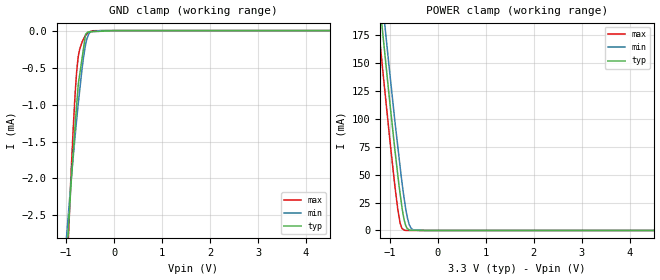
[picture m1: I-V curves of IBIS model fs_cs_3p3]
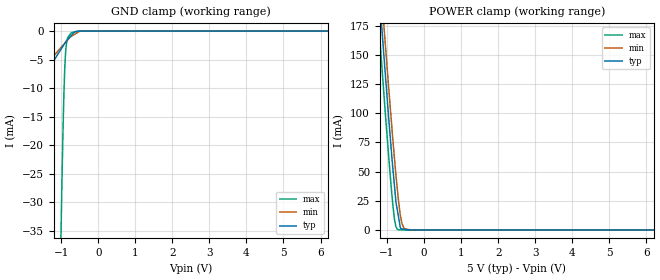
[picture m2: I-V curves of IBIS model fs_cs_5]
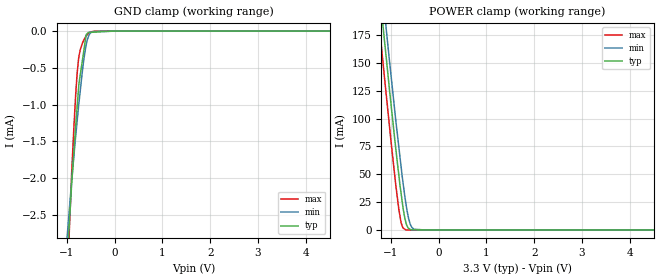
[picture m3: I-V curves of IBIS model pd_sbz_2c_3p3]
|Texas Instruments Incorporated
| 16-Bit 600KSPS Serial ADC with Ref and Pseudo Bipolar,
| Fully Differential Input
| Marketing part#   Digital Voltage Range   Package-type   #pins
| ADS8372IBRHPR   2.7V - 5.25V   VQFN   28
| ADS8372IBRHPRG4   2.7V - 5.25V   VQFN   28
| ADS8372IBRHPT   2.7V - 5.25V   VQFN   28
| ADS8372IBRHPTG4   2.7V - 5.25V   VQFN   28
| ADS8372IRHPR   2.7V - 5.25V   VQFN   28
| ADS8372IRHPRG4   2.7V - 5.25V   VQFN   28
| ADS8372IRHPT   2.7V - 5.25V   VQFN   28
| ADS8372IRHPTG4   2.7V - 5.25V   VQFN   28
[IBIS Ver]   3.2
[File name]   ads8372.ibs
|SIMDE Ver   V3.0 - 201101 - RHL4 - Build 457
[File Rev]   1.0
[Date]   6/17/2011
[Source]
| Texas Instruments Incorporated.
| Analog-eLab Design Center, HPA
| 12500 TI Blvd
| Dallas, TX -75243
| e-mail: elab_scm_ibis@list.ti.com
[Notes]   Revision History:
| Rev 1.0: 6/17/2011
| - Initial version of the model
| - Model generated from simulations in TISPICE
| - Model matched to SPICE simulation
| - C_comp although listed in numerical order of value are
|   obtained from varying PVT conditions. For PVT conditions for
|   each specific value refer the buffer description under
|   respective [Model]. IBIS model user is responsible for using
|   appropriate C_comp to simulate for Signal Integrity.
| - Model names with a trailing _3p3 contains the model for
|   3.3V [3.0V and 3.6V]. Model names with a trailing _5 contains
|   the model for 5.0V [4.75V and 5.25V].
| - SDO pin ibis is modeled in two modes of operation sdo_1drv_*
|   with single driver & sdo_2drv_* 2 driver blocks connected to SDO pad pin.
|   Inbuilt OR logic is used for mode selection.
| - Relative part of ADS8380.
[Disclaimer]
| This model is designed as an aid for customers of Texas Instruments.
| TI and its licensors and suppliers make no warranties, either expressed
| or implied, with respect to this  model, including the warranties of
| merchantability or fitness for a particular purpose. The model is
| provided solely on an "as is" basis. The entire risk as to its quality
| and performance is with the customer.
[Copyright]
 (C) Copyright 2011 Texas Instruments Incorporated.All rights reserved.
|   ADS8372
[Component]   ADS8372
[Manufacturer]   TI
[Package]   |28 VQFN   -  RHP package
|   typ   min   max
R_pkg   0.07673   0.07403   0.08176
L_pkg   1.23150nH   1.17718nH   1.32308nH
C_pkg   0.19965pF   0.19514pF   0.20511pF
[Pin]  signal_name   model_name   R_pin   L_pin   C_pin
1   AGND   GND   0.07820   1.25848nH  0.20073pF
2   AGND   GND   0.07674   1.23138nH  0.20002pF
3   +VA   POWER   0.07537   1.20618nH  0.19911pF
4   AGND   GND   0.07406   1.18248nH  0.19804pF
5   AGND   GND   0.07441   1.18988nH  0.19838pF
6   +VA   POWER   0.07613   1.22288nH  0.20045pF
7   REFM   GND   0.08029   1.30198nH  0.20374pF
8   REFIN   TERM   0.07725   1.24688nH  0.19750pF
9   REFOUT   TERM   0.07703   1.24278nH  0.19851pF
10   NC   NC   0.07445   1.19468nH  0.19621pF
11   +IN   TERM   0.07407   1.18748nH  0.19545pF
12   -IN   TERM   0.07475   1.20008nH  0.19514pF
13   NC   NC   0.00007   0.00128nH  0.12029pF
14   +VA   POWER   0.08623   1.41618nH  0.20518pF
15   AGND   GND   0.07587   1.21778nH  0.19615pF
16   +VA   POWER   0.07435   1.18858nH  0.19555pF
17   +VA   POWER   0.07401   1.18158nH  0.19546pF
18   AGND   GND   0.07505   1.20028nH  0.19719pF
19   AGND   GND   0.03811   0.83717nH  0.23761pF
20   +VBD   POWER   0.07794   1.25358nH  0.19975pF
21   BDGND   GND   0.07776   1.25028nH  0.19781pF
22   BUSY   BUSY   0.08176   1.32308nH  0.20511pF
23   SDO   SDO   0.07780   1.24828nH  0.20181pF
24   SCLK   SCLK_CONVEST   0.07628   1.21958nH  0.20091pF
25   _CONVST   SCLK_CONVEST   0.07403   1.17718nH  0.19891pF
26   _CS   FS_CS   0.07482   1.19198nH  0.19852pF
27   FS   FS_CS   0.07568   1.20828nH  0.20001pF
28   PD   PD_SBZ_2C   0.08058   1.30088nH  0.20427pF
29   THERMAL_PAD   NC   0.00007   0.00128nH  2.20537pF
|   Model Selectors
[Model Selector] FS_CS
fs_cs_3p3  3.3V digital input
fs_cs_5   5.0V digital input
[Model Selector] PD_SBZ_2C
pd_sbz_2c_3p3  3.3V digital input
pd_sbz_2c_5   5.0V digital input
[Model Selector] SCLK_CONVEST
sclk_convest_3p3  3.3V digital input
sclk_convest_5   5.0V digital input
[Model Selector] BUSY
busy_3p3  3.3V digital 3-state
busy_5   5.0V digital 3-state
[Model Selector] SDO
sdo_1drv_3p3  3.3V digital 3-state
sdo_1drv_5   5.0V digital 3-state
sdo_2drv_3p3  3.3V digital 3-state
sdo_2drv_5   5.0V digital 3-state
[Model Selector] TERM
term_3-3V  3.3V nominal termination
term_5-0V  5.0V nominal termination
[Model] term_3-3V
Model_type Terminator
C_comp   1.0e-20F  1.0e-20F  1.0e-20F
|   typ   min   max
[Voltage Range]   3.3V   3.0V   3.6V
[POWER Clamp Reference]   3.3V   3.0V   3.6V
[GND Clamp Reference]   0V   0V   0V
|Ambient Temperature   25   85   -40
|Junction Temperature
[Temperature Range]   35   95   -40
[Model] term_5-0V
Model_type Terminator
C_comp   1.0e-20F  1.0e-20F  1.0e-20F
|   typ   min   max
[Voltage Range]   5.0V   4.75V   5.25V
[POWER Clamp Reference]   5.0V   4.75V   5.25V
[GND Clamp Reference]   0V   0V   0V
|Ambient Temperature   25   85   -40
|Junction Temperature
[Temperature Range]   35   95   -40
| Models and submodels in the file (14): fs_cs_3p3 (Input), fs_cs_5 (Input), pd_sbz_2c_3p3 (Input), pd_sbz_2c_5 (Input), sclk_convest_3p3 (Input), sclk_convest_5 (Input), busy_3p3 (3-state), busy_5 (3-state), sdo_1drv_3p3 (3-state), sdo_1drv_5 (3-state), sdo_2drv_3p3 (3-state), sdo_2drv_5 (3-state), term_3-3V (Terminator), term_5-0V (Terminator)
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|   fs_cs_3p3 Model
[Model]   fs_cs_3p3
Model_type   Input
Vinl = 0.8
Vinh = 2.3
|   typ   min   max
|   (nom PVT)   (fast PVT)   (slow PVT)
|C_comp from frequency sweep method (F=40MHz)
|Average
C_comp   9.345e-13   8.948e-13   9.802e-13
|C_comp from LC tank measurement(L=1nH)
|Average
|Resonant Frequency(Hz)   6.530e+09   6.860e+09   6.210e+09
|C_comp   5.946e-13   5.388e-13   6.575e-13
| Where nom  PVT is Nominal Process, 3.3V, 35C
|   Fast PVT is Strong Process,  3.6V, -40C
|   Slow PVT is Weak Process,   3V, 95C
[Model Spec]
Vinl   0.8   0.8   0.8
Vinh   2.3   2.0   2.6
[Voltage Range]   3.3   3   3.6
|Ambient Temperature   25   85   -40
|Junction Temperature
[Temperature Range]   35   95   -40
[Power Clamp Reference]   3.3   3   3.6
[GND Clamp Reference]   0   0   0
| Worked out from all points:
|   GND clamp passes 1 mA (typ) near -0.78 V on its own axis
|   POWER clamp passes 1 mA (typ) near -0.61 V on its own axis
[GND Clamp]
|   Voltage   I(typ)   I(min)   I(max)
-3.3V     -29.5mA    -22.08mA   -346.9mA
-1.48V    -8.435mA   -6.749mA   -11.2mA
-897.6mV  -2.079mA   -2.033mA   -1.938mA
-813.6mV  -1.291mA   -1.432mA   -869.3uA
-781.2mV  -1.016mA   -1.213mA   -563uA
-752.4mV  -772.5uA   -1.02mA    -377.4uA
-666mV    -368uA     -504.3uA   -154.1uA
-594mV    -49.28uA   -188.5uA   -63.98uA
-547.8mV  -18.81uA   -78.25uA   -34.03uA
-483mV    -16.57uA   -13.84uA   -10.13uA
-285mV    -9.73uA    -61.45nA   -1.03uA
6.6V      0A         0A         0A
[POWER Clamp]
|   Voltage   I(typ)   I(min)   I(max)
-3.3V     1.135A     1.155A     1.11A
-1.318V   249.1mA    274.8mA    216.8mA
-1.176V   187.9mA    213.6mA    155.3mA
-1.13V    168.7mA    194.3mA    135.5mA
-1.023V   123.4mA    149.3mA    90.46mA
-896.4mV  72.45mA    98.1mA     40mA
-835.2mV  49.7mA     75.13mA    19.03mA
-784.8mV  32.38mA    56.22mA    6.372mA
-691.2mV  7.748mA    25.44mA    159.7uA
-597mV    508.4uA    5.363mA    2.122uA
-516mV    127uA      660uA      747.1nA
6.6V      0A         0A         0A
|   fs_cs_5 Model
[Model]   fs_cs_5
Model_type   Input
Vinl = 0.8
Vinh = 4.0
|   typ   min   max
|   (nom PVT)   (fast PVT)   (slow PVT)
|C_comp from frequency sweep method (F=40MHz)
|Average
C_comp   9.085e-13   8.893e-13   9.134e-13
|C_comp from LC tank measurement(L=1nH)
|Average
|Resonant Frequency(Hz)   6.870e+09   7.150e+09   6.610e+09
|C_comp   5.372e-13   4.960e-13   5.803e-13
| Where nom  PVT is Nominal Process, 5V, 35C
|   Fast PVT is Strong Process,  5.25V, -40C
|   Slow PVT is Weak Process,   4.75V, 95C
[Model Spec]
Vinl   0.8   0.8   0.8
Vinh   4.0   3.75   4.25
[Voltage Range]   5   4.75   5.25
|Ambient Temperature   25   85   -40
|Junction Temperature
[Temperature Range]   35   95   -40
[Power Clamp Reference]   5   4.75   5.25
[GND Clamp Reference]   0   0   0
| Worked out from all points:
|   GND clamp passes 1 mA (typ) near -0.76 V on its own axis
|   POWER clamp passes 1 mA (typ) near -0.62 V on its own axis
[GND Clamp]
|   Voltage   I(typ)   I(min)   I(max)
-5V       -51.14mA   -37.96mA   -1.888A
-4.75V    -47.95mA   -35.65mA   -1.771A
-4.21V    -41.13mA   -30.65mA   -1.516A
-3.533V   -32.56mA   -24.38mA   -1.198A
-2.67V    -21.64mA   -16.53mA   -792.8mA
-1.008V   -3.206mA   -2.891mA   -36.15mA
-939.7mV  -2.519mA   -2.392mA   -14.05mA
-892.5mV  -2.043mA   -2.046mA   -4.874mA
-829.5mV  -1.508mA   -1.585mA   -1.265mA
-729.8mV  -784.8uA   -924.3uA   -289.8uA
-503.5mV  -20.08uA   -23.98uA   -21.48uA
10V       0A         0A         0A
[POWER Clamp]
|   Voltage   I(typ)   I(min)   I(max)
-5V       1.905A     1.922A     1.884A
-1.302V   242mA      267.3mA    209.7mA
-1.126V   166.8mA    192.3mA    134.1mA
-1.08V    147.2mA    173.1mA    114.4mA
-955.5mV  95.9mA     121.9mA    62.77mA
-834.7mV  49.93mA    74.38mA    18.9mA
-761.2mV  24.49mA    47.49mA    2.961mA
-698.3mV  12.62mA    27.18mA    218.3uA
-640mV    1.834mA    12.45mA    14.73uA
-598.5mV  870.6uA    5.545mA    1.881uA
-356.3mV  494.1nA    6.232uA    1.12uA
10V       0A         0A         0A
|   pd_sbz_2c_3p3 Model
[Model]   pd_sbz_2c_3p3
Model_type   Input
Vinl = 0.8
Vinh = 2.3
|   typ   min   max
|   (nom PVT)   (fast PVT)   (slow PVT)
|C_comp from frequency sweep method (F=40MHz)
|Average
C_comp   9.314e-13   9.057e-13   9.837e-13
|C_comp from LC tank measurement(L=1nH)
|Average
|Resonant Frequency(Hz)   6.540e+09   6.860e+09   6.220e+09
|C_comp   5.928e-13   5.388e-13   6.554e-13
| Where nom  PVT is Nominal Process, 3.3V, 35C
|   Fast PVT is Strong Process,  3.6V, -40C
|   Slow PVT is Weak Process,   3V, 95C
[Model Spec]
Vinl   0.8   0.8   0.8
Vinh   2.3   2.0   2.6
[Voltage Range]   3.3   3   3.6
|Ambient Temperature   25   85   -40
|Junction Temperature
[Temperature Range]   35   95   -40
[Power Clamp Reference]   3.3   3   3.6
[GND Clamp Reference]   0   0   0
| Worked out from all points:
|   GND clamp passes 1 mA (typ) near -0.78 V on its own axis
|   POWER clamp passes 1 mA (typ) near -0.61 V on its own axis
[GND Clamp]
|   Voltage   I(typ)   I(min)   I(max)
-3.3V     -29.5mA    -22.08mA   -346.9mA
-1.48V    -8.435mA   -6.749mA   -11.2mA
-897.6mV  -2.079mA   -2.033mA   -1.938mA
-813.6mV  -1.291mA   -1.432mA   -869.3uA
-781.2mV  -1.016mA   -1.213mA   -563uA
-752.4mV  -772.5uA   -1.02mA    -377.4uA
-666mV    -368uA     -504.3uA   -154.1uA
-594mV    -49.28uA   -188.5uA   -63.98uA
-547.8mV  -18.81uA   -78.25uA   -34.03uA
-483mV    -16.57uA   -13.84uA   -10.13uA
-285mV    -9.73uA    -61.45nA   -1.03uA
6.6V      0A         0A         0A
[POWER Clamp]
|   Voltage   I(typ)   I(min)   I(max)
-3.3V     1.135A     1.155A     1.11A
-1.318V   249.1mA    274.8mA    216.8mA
-1.176V   187.9mA    213.6mA    155.3mA
-1.13V    168.7mA    194.3mA    135.5mA
-1.023V   123.4mA    149.3mA    90.46mA
-896.4mV  72.45mA    98.1mA     40mA
-835.2mV  49.7mA     75.13mA    19.03mA
-784.8mV  32.38mA    56.22mA    6.372mA
-691.2mV  7.748mA    25.44mA    159.7uA
-597mV    508.4uA    5.363mA    2.122uA
-516mV    127uA      660uA      747.1nA
6.6V      0A         0A         0A
